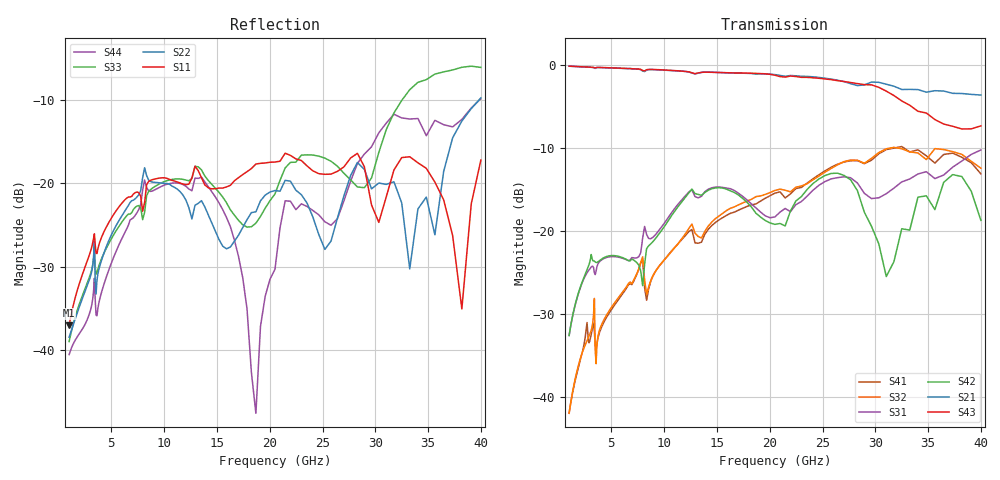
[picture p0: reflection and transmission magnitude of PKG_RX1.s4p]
! Created Mon Sep 18 16:18:19 2017
# hz S ma R 50
! 4 Port Network Data from SP1.SP block
! freq  magS11  angS11  magS12  angS12  magS13  angS13  magS14  angS14
!  magS21  angS21  magS22  angS22  magS23  angS23  magS24  angS24
!  magS31  angS31  magS32  angS32  magS33  angS33  magS34  angS34
!  magS41  angS41  magS42  angS42  magS43  angS43  magS44  angS44
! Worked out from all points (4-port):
!   161 points, 1 GHz to 40 GHz, reference 50 ohm
!   strongest paths, dB at 1 GHz, 2.515 GHz, 6.325 GHz, 15.91 GHz, 40 GHz:
!     S43: -0.1, -0.2, -0.4, -0.9, -7.3
!     S21: -0.1, -0.2, -0.4, -0.9, -3.6
!     S42: -32.6, -25.3, -23.4, -14.9, -18.7
!     S31: -32.6, -25.5, -23.4, -14.8, -10.2
!     S32: -42.0, -33.8, -26.9, -17.5, -12.4
!     S41: -42.0, -32.9, -27.1, -18.1, -13.1
!   lowest |S11| = -37.0 dB at 1 GHz (marker M1), VSWR 1.03, Z = 51.3 + j0.626 ohm
!   |S11| at or under -10 dB: start of sweep to end of sweep
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1e9  0.01414 25.6  0.9885 -18.0  0.02342 74.6  0.007942 -111.9
     0.9885 -18.0  0.01197 47.9  0.007969 -111.9  0.02344 66.8
     0.02342 74.6  0.007969 -111.9  0.01128 19.3  0.989 -17.3
     0.007942 -111.9  0.02344 66.8  0.989 -17.3  0.009425 38.3
1.002969e10  0.1081 -113.4  0.9352 -176.0  0.1118 40.2  0.06712 109.1
             0.9352 -176.0  0.09996 -57.5  0.06704 101.0  0.1067 157.0
             0.1118 40.2  0.06704 101.0  0.1027 -108.5  0.938 -169.1
             0.06712 109.1  0.1067 157.0  0.938 -169.1  0.09784 -50.6
1.869111e10  0.1307 -127.4  0.8853 32.6  0.1382 -31.2  0.1457 -44.8
             0.8853 32.6  0.0676 8.7  0.1613 -60.5  0.1282 -67.4
             0.1382 -31.2  0.1613 -60.5  0.0578 -126.6  0.8948 44.9
             0.1457 -44.8  0.1282 -67.4  0.8948 44.9  0.004189 -46.7
2.464845e10  0.1144 -153.6  0.8461 -74.1  0.1886 -44.7  0.2183 -147.0
             0.8461 -74.1  0.04938 -88.5  0.2145 -167.6  0.2059 89.9
             0.1886 -44.7  0.2145 -167.6  0.1457 -155.0  0.836 -58.6
             0.2183 -147.0  0.2059 89.9  0.836 -58.6  0.06484 -86.2
3.033231e10  0.05843 -153.1  0.7902 -174.5  0.1588 -145.8  0.2927 101.4
             0.7902 -174.5  0.1005 -116.4  0.2978 78.0  0.08368 -51.4
             0.1588 -145.8  0.2978 78.0  0.1533 -137.9  0.7367 -163.1
             0.2927 101.4  0.08368 -51.4  0.7367 -163.1  0.201 -86.1
3.819744e10  0.0177 -106.8  0.6765 45.0  0.2646 70.3  0.2788 -68.1
             0.6765 45.0  0.2365 -11.9  0.2903 -96.8  0.2133 19.9
             0.2646 70.3  0.2903 -96.8  0.4968 78.2  0.4132 76.6
             0.2788 -68.1  0.2133 19.9  0.4132 76.6  0.2419 44.6
4e10  0.1381 -100.4  0.6619 10.2  0.3086 50.7  0.2214 -106.8
      0.6619 10.2  0.3256 -53.7  0.2396 -134.4  0.1161 -27.3
      0.3086 50.7  0.2396 -134.4  0.4957 44.0  0.4312 53.8
      0.2214 -106.8  0.1161 -27.3  0.4312 53.8  0.3218 -25.2
